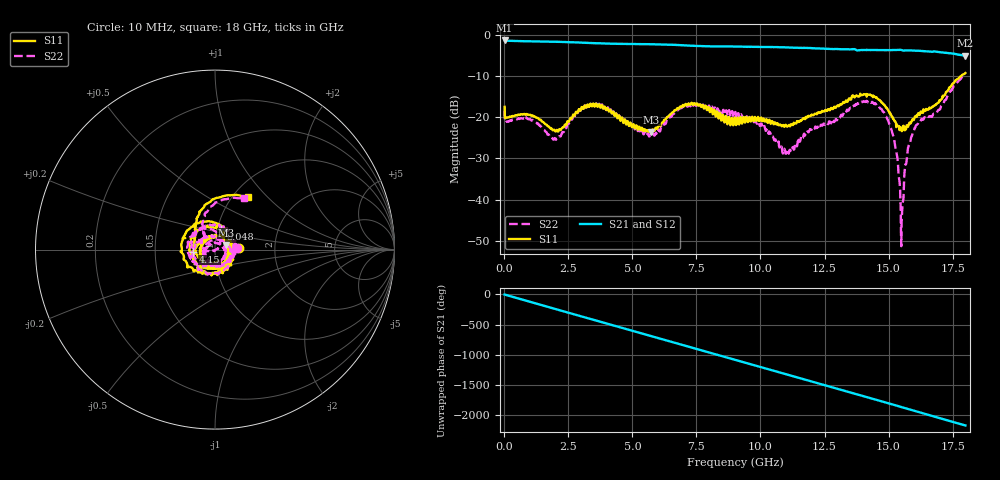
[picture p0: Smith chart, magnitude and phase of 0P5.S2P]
!Agilent Technologies,E5071C,MY46316741,A.11.02
!Date: Tue Sep 22 10:33:01 2020
!Data & Calibration Information:
!Freq	S11:SOLT4(ON)	S21:SOLT4(ON)	S12:SOLT4(ON)	S22:SOLT4(ON)
!PortZ  Port1:50+j0  Port2:50+j0
!Above PortZ is port z conversion or system Z0 setting when saving the data.
!When reading, reference impedance value at option line is always used.
# Hz S dB R 50
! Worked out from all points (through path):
!   1561 points, 10 MHz to 18 GHz, reference 50 ohm
!   highest |S21| = -1.39 dB at 10 MHz (marker M1); lowest = -5.1 dB at 18 GHz (marker M2)
!   group delay of S21, straight-line fit = 335 ps
!   lowest |S11| = -23.6 dB at 5.741 GHz (marker M3), VSWR 1.14, Z = 56.4 + j2.86 ohm
!   |S11| at or under -10 dB: start of sweep to 17.84 GHz
!   |S22| runs from -51.3 to -9.7 dB; largest |S21 - S12| = 0.022
!   S11 on the Smith chart (normalised r, x): 10 MHz: 1.31, +0.02; 4.15 GHz: 0.79, -0.02; 8.048 GHz: 1.03, +0.24; 18 GHz: 1.17, +0.77
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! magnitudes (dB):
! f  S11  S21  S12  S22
! 10 MHz  -17.5  -1.4  -1.4  -18.4
! 1.059 GHz  -19.6  -1.6  -1.6  -20.8
! 1.97 GHz  -23.3  -1.7  -1.7  -25.1
! 3.02 GHz  -17.5  -1.9  -1.9  -17.7
! 4.15 GHz  -18.4  -2.2  -2.2  -18.1
! 5.741 GHz  -23.6  -2.3  -2.3  -24.6
! 6.007 GHz  -22.2  -2.3  -2.4  -23.3
! 6.918 GHz  -17.6  -2.5  -2.6  -17.8
! 8.048 GHz  -18.5  -2.8  -2.8  -18.1
! 9.005 GHz  -20.2  -2.9  -2.9  -18.8
! 9.974 GHz  -20.7  -3.0  -3.0  -22.1
! 10.93 GHz  -22.3  -3.1  -3.1  -27.7
! 12.01 GHz  -19.4  -3.2  -3.3  -22.6
! 14.08 GHz  -14.5  -3.7  -3.7  -16.3
! 15 GHz  -18.5  -3.7  -3.8  -21.1
! 15.29 GHz  -21.4  -3.7  -3.8  -28.1
! 15.46 GHz  -22.5  -3.6  -3.7  -40.0
! 15.52 GHz  -23.4  -3.7  -3.7  -43.7
! 15.71 GHz  -22.0  -3.8  -3.7  -30.6
! 16.02 GHz  -20.1  -3.9  -3.9  -22.6
! 16.93 GHz  -16.5  -4.2  -4.3  -18.4
! 18 GHz  -9.3  -5.1  -5.1  -9.7
